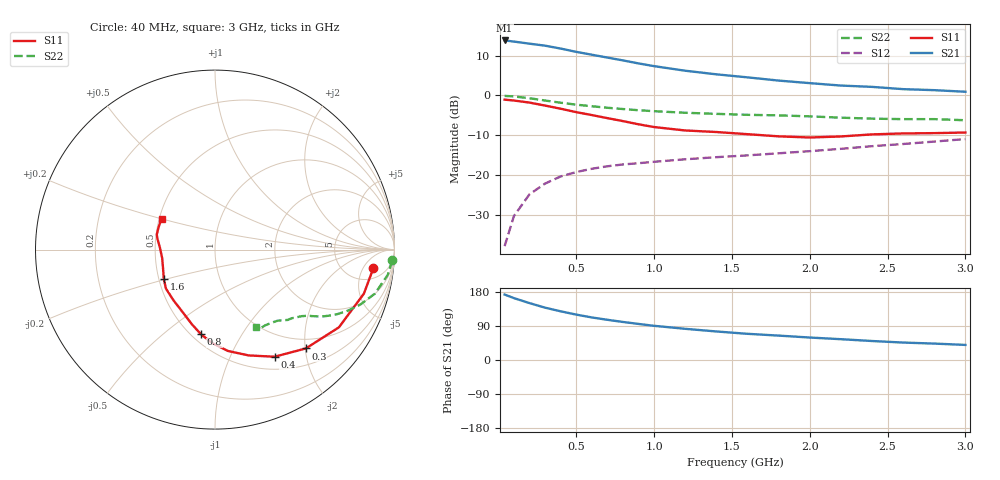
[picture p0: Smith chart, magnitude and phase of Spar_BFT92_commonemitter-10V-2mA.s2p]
! Filename:  BFT92F.S2P  Version:  2.0
! NXP part #: BFT92  Date: May 1990
! Bias condition: Vce=-10V, Ic=-2mA
#  MHz  S  MA  R  50
! Freq  S11  S21  S12  S22  !GUM [dB]
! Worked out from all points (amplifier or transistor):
!   21 points, 40 MHz to 3 GHz, reference 50 ohm
!   highest |S21| = 13.8 dB at 40 MHz (marker M1)
!   |S21| within 3 dB of that: start of sweep to 520.5 MHz
!   unconditionally stable (mu >= 1): 1.546 GHz to end of sweep
!   at 300 MHz: K = 0.33, MSG = 17.3 dB, |S12| = -22.0 dB
!   at 1 GHz: K = 0.81, MSG = 12.0 dB, |S12| = -16.6 dB
!   at 3 GHz: K = 1.05, MAG = 4.6 dB, |S12| = -10.9 dB
!   S11 on the Smith chart (normalised r, x): 40 MHz: 8, -8; 300 MHz: 0.81, -2.01; 400 MHz: 0.67, -1.49; 800 MHz: 0.56, -0.68; 1.6 GHz: 0.53, -0.19; 3 GHz: 0.51, +0.20
40  0.888 -6.8  4.886 172.7  0.013 85.3  0.989 -3.5
100  0.865 -16.5  4.731 163.3  0.031 79.3  0.973 -8.3
200  0.815 -32.1  4.453 150.1  0.058 70.9  0.924 -15.4
300  0.748 -47.4  4.204 138.1  0.079 64.4  0.865 -20.8
400  0.683 -60.9  3.868 128.5  0.097 59.5  0.812 -24.9
500  0.619 -72.3  3.518 119.8  0.11 56.1  0.768 -28.0
600  0.569 -82.8  3.24 112.3  0.121 53.4  0.734 -30.1
700  0.521 -91.7  2.984 106.1  0.13 51.7  0.702 -32.1
800  0.478 -99.4  2.75 100.4  0.137 50.8  0.677 -33.3
900  0.436 -107.1  2.521 95.2  0.142 50.1  0.654 -34.5
1000  0.403 -114.3  2.331 90.2  0.148 49.8  0.636 -35.4
1200  0.365 -129.4  2.042 82.3  0.159 49.8  0.608 -37.6
1400  0.349 -141.6  1.841 75.3  0.169 50.5  0.589 -39.9
1600  0.328 -150.5  1.687 69.1  0.178 52.4  0.573 -41.9
1800  0.308 -160.0  1.537 64.4  0.189 54.1  0.564 -44.0
2000  0.298 -170.9  1.428 59.3  0.201 55.8  0.548 -45.9
2200  0.307 178.0  1.332 54.9  0.215 57.3  0.528 -48.6
2400  0.326 169.5  1.282 50.1  0.232 58.4  0.513 -53.0
2600  0.335 165.5  1.201 46.0  0.247 59.6  0.506 -56.7
2800  0.338 158.6  1.166 43.3  0.265 60.9  0.506 -59.8
3000  0.344 149.8  1.114 39.8  0.285 61.6  0.49 -62.2
